(* Received SV array buffer *)
TYPE ST_SVBUFFER_IED_MUnn_LLN0_MSVCB02 : 
STRUCT
	index: UINT(0..cArrayBufferSize_IED_MUnn_LLN0_MSVCB02_Asdu1-1) := 0; (* Index of next free array element *)
	
	IED_MUnn_InnATCTR1_AmpSv_instMag_i: ARRAY [0..cArrayBufferSize_IED_MUnn_LLN0_MSVCB02_Asdu1-1] OF DINT;
	IED_MUnn_InnATCTR1_AmpSv_q: ARRAY [0..cArrayBufferSize_IED_MUnn_LLN0_MSVCB02_Asdu1-1] OF ST_AcsiQuality;
	IED_MUnn_InnBTCTR2_AmpSv_instMag_i: ARRAY [0..cArrayBufferSize_IED_MUnn_LLN0_MSVCB02_Asdu1-1] OF DINT;
	IED_MUnn_InnBTCTR2_AmpSv_q: ARRAY [0..cArrayBufferSize_IED_MUnn_LLN0_MSVCB02_Asdu1-1] OF ST_AcsiQuality;
	IED_MUnn_InnCTCTR3_AmpSv_instMag_i: ARRAY [0..cArrayBufferSize_IED_MUnn_LLN0_MSVCB02_Asdu1-1] OF DINT;
	IED_MUnn_InnCTCTR3_AmpSv_q: ARRAY [0..cArrayBufferSize_IED_MUnn_LLN0_MSVCB02_Asdu1-1] OF ST_AcsiQuality;
	IED_MUnn_InnNTCTR4_AmpSv_instMag_i: ARRAY [0..cArrayBufferSize_IED_MUnn_LLN0_MSVCB02_Asdu1-1] OF DINT;
	IED_MUnn_InnNTCTR4_AmpSv_q: ARRAY [0..cArrayBufferSize_IED_MUnn_LLN0_MSVCB02_Asdu1-1] OF ST_AcsiQuality;
	IED_MUnn_UnnATVTR1_VolSv_instMag_i: ARRAY [0..cArrayBufferSize_IED_MUnn_LLN0_MSVCB02_Asdu1-1] OF DINT;
	IED_MUnn_UnnATVTR1_VolSv_q: ARRAY [0..cArrayBufferSize_IED_MUnn_LLN0_MSVCB02_Asdu1-1] OF ST_AcsiQuality;
	IED_MUnn_UnnBTVTR2_VolSv_instMag_i: ARRAY [0..cArrayBufferSize_IED_MUnn_LLN0_MSVCB02_Asdu1-1] OF DINT;
	IED_MUnn_UnnBTVTR2_VolSv_q: ARRAY [0..cArrayBufferSize_IED_MUnn_LLN0_MSVCB02_Asdu1-1] OF ST_AcsiQuality;
	IED_MUnn_UnnCTVTR3_VolSv_instMag_i: ARRAY [0..cArrayBufferSize_IED_MUnn_LLN0_MSVCB02_Asdu1-1] OF DINT;
	IED_MUnn_UnnCTVTR3_VolSv_q: ARRAY [0..cArrayBufferSize_IED_MUnn_LLN0_MSVCB02_Asdu1-1] OF ST_AcsiQuality;
	IED_MUnn_UnnNTVTR4_VolSv_instMag_i: ARRAY [0..cArrayBufferSize_IED_MUnn_LLN0_MSVCB02_Asdu1-1] OF DINT;
	IED_MUnn_UnnNTVTR4_VolSv_q: ARRAY [0..cArrayBufferSize_IED_MUnn_LLN0_MSVCB02_Asdu1-1] OF ST_AcsiQuality;
END_STRUCT
END_TYPE
